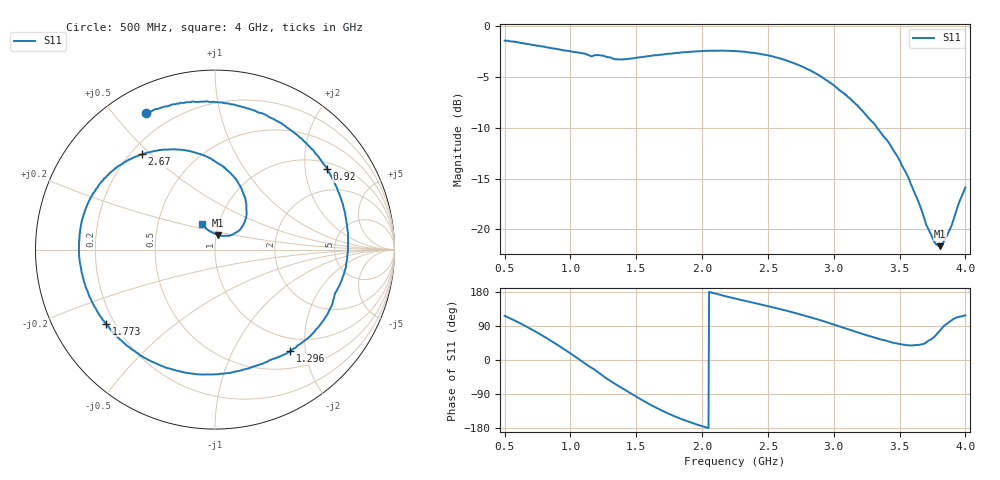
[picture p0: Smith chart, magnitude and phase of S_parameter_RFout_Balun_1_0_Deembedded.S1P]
!Agilent Technologies,E5071B,MY42403504,A.06.51
!Date: Wed Feb 26 14:54:27 2014
!Data & Calibration Information:
!Freq	S11:SOLT1(ON)
# Hz S dB R 50
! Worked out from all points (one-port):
!   801 points, 500 MHz to 4 GHz, reference 50 ohm
!   lowest |S11| = -21.6 dB at 3.808 GHz (marker M1), VSWR 1.18, Z = 51.1 + j8.33 ohm
!   |S11| at or under -10 dB: 3.33 GHz to end of sweep
!   S11 on the Smith chart (normalised r, x): 500 MHz: 0.11, +0.61; 920 MHz: 1.20, +2.62; 1.296 GHz: 0.76, -1.72; 1.773 GHz: 0.17, -0.30; 2.67 GHz: 0.24, +0.47; 4 GHz: 0.83, +0.24
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5e8  -1.40 116.8
6.09375e8  -1.57 98.6
7.14375e8  -1.84 79.0
8.15e8  -2.06 58.7
9.2e8  -2.30 35.7
9.375e8  -2.33 31.7
1.025e9  -2.52 11.4
1.10375e9  -2.66 -7.6
1.2e9  -2.82 -29.8
1.29625e9  -3.05 -53.6
1.375e9  -3.27 -70.7
1.4625e9  -3.16 -88.8
1.55e9  -3.03 -106.8
1.655e9  -2.86 -126.5
1.773125e9  -2.67 -145.9
1.8125e9  -2.61 -151.6
2.009375e9  -2.44 -175.6
2.25e9  -2.43 162.3
2.45125e9  -2.74 146.1
2.67e9  -3.50 127.5
2.6875e9  -3.58 125.9
2.8975e9  -4.88 105.0
3.125e9  -7.12 79.6
3.330625e9  -10.00 57.0
3.5625e9  -14.76 38.8
3.715625e9  -19.91 50.0
3.8075e9  -21.64 77.9
4e9  -15.86 117.7
